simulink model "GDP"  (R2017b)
settings: Solver=FixedStepDiscrete  StartTime=0.0  StopTime=10.0  FixedStep=0.01  RelTol=1e-3  EnableMultiTasking=on
undefined symbols (not defined in the file): ASWTYPE_FALSE, ASWTYPE_TRUE, CcGDP_DCCANBusOffFltTi_ms, Enum_DCCDCConnSt, Enum_LDPCC2St, GDP_CONST1_NUMB, GDP_RUNTIME_MS
libraries: AIWAYS_Powertrain_BMS_lib x68
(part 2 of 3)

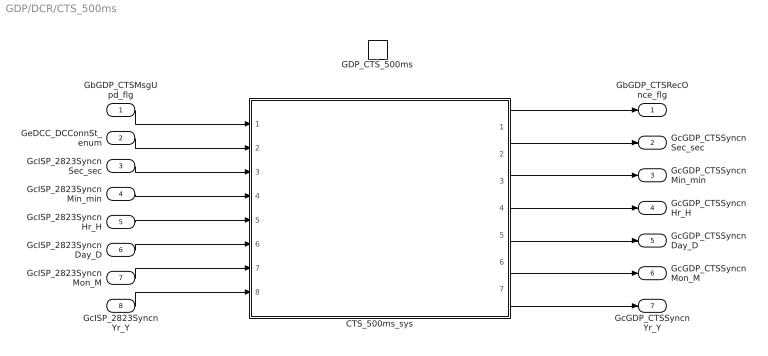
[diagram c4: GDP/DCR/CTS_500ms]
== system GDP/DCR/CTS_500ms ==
  GbGDP_CTSMsgUpd_flg : Inport
  GeDCC_DCConnSt_enum : Inport  Port=2
  GcISP_2823SyncnSec_sec : Inport  Port=3
  GcISP_2823SyncnMin_min : Inport  Port=4
  GcISP_2823SyncnHr_H : Inport  Port=5
  GcISP_2823SyncnDay_D : Inport  Port=6
  GcISP_2823SyncnMon_M : Inport  Port=7
  GcISP_2823SyncnYr_Y : Inport  Port=8
  GDP_CTS_500ms : TriggerPort  TriggerType=function-call  VariantControl=(inherit)
  CTS_500ms_sys : Subsystem
  GbGDP_CTSRecOnce_flg : Outport
  GcGDP_CTSSyncnSec_sec : Outport  Port=2
  GcGDP_CTSSyncnMin_min : Outport  Port=3
  GcGDP_CTSSyncnHr_H : Outport  Port=4
  GcGDP_CTSSyncnDay_D : Outport  Port=5
  GcGDP_CTSSyncnMon_M : Outport  Port=6
  GcGDP_CTSSyncnYr_Y : Outport  Port=7
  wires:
  GbGDP_CTSMsgUpd_flg/1 -> CTS_500ms_sys/1(GbGDP_CTSMsgUpd_flg)
  GeDCC_DCConnSt_enum/1 -> CTS_500ms_sys/2(GeDCC_DCConnSt_enum)
  GcISP_2823SyncnSec_sec/1 -> CTS_500ms_sys/3(GcISP_2823SyncnSec_sec)
  GcISP_2823SyncnMin_min/1 -> CTS_500ms_sys/4(GcISP_2823SyncnMin_min)
  GcISP_2823SyncnHr_H/1 -> CTS_500ms_sys/5(GcISP_2823SyncnHr_H)
  GcISP_2823SyncnDay_D/1 -> CTS_500ms_sys/6(GcISP_2823SyncnDay_D)
  GcISP_2823SyncnMon_M/1 -> CTS_500ms_sys/7(GcISP_2823SyncnMon_M)
  GcISP_2823SyncnYr_Y/1 -> CTS_500ms_sys/8(GcISP_2823SyncnYr_Y)
  CTS_500ms_sys/1(GbGDP_CTSRecOnce_flg) -> GbGDP_CTSRecOnce_flg/1
  CTS_500ms_sys/2(GcGDP_CTSSyncnSec_sec) -> GcGDP_CTSSyncnSec_sec/1
  CTS_500ms_sys/3(GcGDP_CTSSyncnMin_min) -> GcGDP_CTSSyncnMin_min/1
  CTS_500ms_sys/4(GcGDP_CTSSyncnHr_H) -> GcGDP_CTSSyncnHr_H/1
  CTS_500ms_sys/5(GcGDP_CTSSyncnDay_D) -> GcGDP_CTSSyncnDay_D/1
  CTS_500ms_sys/6(GcGDP_CTSSyncnMon_M) -> GcGDP_CTSSyncnMon_M/1
  CTS_500ms_sys/7(GcGDP_CTSSyncnYr_Y) -> GcGDP_CTSSyncnYr_Y/1

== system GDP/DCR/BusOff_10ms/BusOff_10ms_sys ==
  GbISP_DCCANBusOffFlt_flg : Inport
  GbISP_DCChrgCanNetStatus_flg : Inport  Port=2
  Constant : Constant  Value=GDP_RUNTIME_MS
  Constant1 : Constant  Value=CcGDP_DCCANBusOffFltTi_ms
  Delay : AIWAYS_Powertrain_BMS_lib/Debounce & Delay/BMSDelay
  GDP_GbISP_DCCANBusOffFlt_flg : AIWAYS_Powertrain_BMS_lib/Signals/OverWrite  OverWrite_Value=CbGDP_DCCANBusOffFltOvr_flg  OverWrite_flag=CbGDP_DCCANBusOffFltOvrSwt_flg
  Logical Operator : Logic  AllPortsSameDT=off  OutDataTypeStr=boolean
  GbGDP_DCCANBusOffFlt_flg : Outport
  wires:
  GDP_GbISP_DCCANBusOffFlt_flg/1 -> GbGDP_DCCANBusOffFlt_flg/1  "GbGDP_DCCANBusOffFlt_flg"
  Constant/1 -> Delay/2
  Constant1/1 -> Delay/3
  Delay/1 -> GDP_GbISP_DCCANBusOffFlt_flg/1
  GbISP_DCCANBusOffFlt_flg/1 -> Logical Operator/1  "GbISP_DCCANBusOffFlt_flg"
  GbISP_DCChrgCanNetStatus_flg/1 -> Logical Operator/2  "GbISP_DCChrgCanNetStatus_flg"
  Logical Operator/1 -> Delay/1

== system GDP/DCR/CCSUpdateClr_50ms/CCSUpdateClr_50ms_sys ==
  Constant : Constant  Value=ASWTYPE_FALSE
  GDP_GbGDP_CCSMsgUpd_flg : AIWAYS_Powertrain_BMS_lib/Signals/OverWrite  OverWrite_Value=CbGDP_CCSMsgUpdOvr_flg  OverWrite_flag=CbGDP_CCSMsgUpdOvrSwt_flg
  Signal Conversion1 : SignalConversion  OverrideOpt=off
  GbGDP_CCSMsgUpd_flg : Outport
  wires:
  Constant/1 -> Signal Conversion1/1
  GDP_GbGDP_CCSMsgUpd_flg/1 -> GbGDP_CCSMsgUpd_flg/1  "GbGDP_CCSMsgUpd_flg"
  Signal Conversion1/1 -> GDP_GbGDP_CCSMsgUpd_flg/1

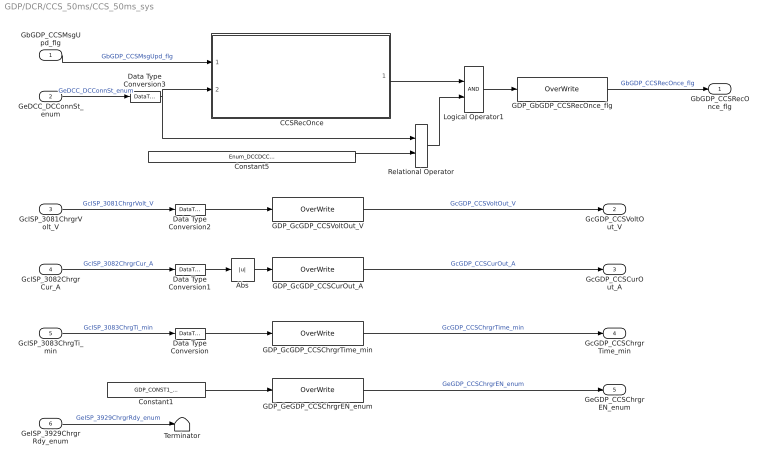
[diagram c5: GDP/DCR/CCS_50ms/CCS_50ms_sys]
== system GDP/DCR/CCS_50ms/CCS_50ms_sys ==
  GbGDP_CCSMsgUpd_flg : Inport
  GeDCC_DCConnSt_enum : Inport  Port=2
  GcISP_3081ChrgrVolt_V : Inport  Port=3
  GcISP_3082ChrgrCur_A : Inport  Port=4
  GcISP_3083ChrgTi_min : Inport  Port=5
  GeISP_3929ChrgrRdy_enum : Inport  Port=6
  " CCSRecOnce" : Subsystem
  Abs : Abs
  Constant1 : Constant  Value=GDP_CONST1_NUMB
  Constant5 : Constant  Value=Enum_DCCDCConnSt.Enum_DCCDCConnSt_Chrging
  Data Type Conversion{,1..3} (4 alike) : DataTypeConversion
  GDP_GbGDP_CCSRecOnce_flg : AIWAYS_Powertrain_BMS_lib/Signals/OverWrite  OverWrite_Value=CbGDP_CCSRecOnceOvr_flg  OverWrite_flag=CbGDP_CCSRecOnceOvrSwt_flg
  GDP_GcGDP_CCSChrgrTime_min : AIWAYS_Powertrain_BMS_lib/Signals/OverWrite  OverWrite_Value=CcGDP_CCSChrgrTimeOvr_min  OverWrite_flag=CbGDP_CCSChrgrTimeOvrSwt_flg
  GDP_GcGDP_CCSCurOut_A : AIWAYS_Powertrain_BMS_lib/Signals/OverWrite  OverWrite_Value=CcGDP_CCSCurOutOvr_A  OverWrite_flag=CbGDP_CCSCurOutOvrSwt_flg
  GDP_GcGDP_CCSVoltOut_V : AIWAYS_Powertrain_BMS_lib/Signals/OverWrite  OverWrite_Value=CcGDP_CCSVoltOutOvr_V  OverWrite_flag=CbGDP_CCSVoltOutOvrSwt_flg
  GDP_GeGDP_CCSChrgrEN_enum : AIWAYS_Powertrain_BMS_lib/Signals/OverWrite  OverWrite_Value=CeGDP_CCSChrgrENOvr_enum  OverWrite_flag=CbGDP_CCSChrgrENOvrSwt_flg
  Logical Operator1 : Logic  AllPortsSameDT=off  OutDataTypeStr=boolean
  Relational Operator : RelationalOperator  Operator===  OutDataTypeStr=boolean
  Terminator : Terminator
  GbGDP_CCSRecOnce_flg : Outport
  GcGDP_CCSVoltOut_V : Outport  Port=2
  GcGDP_CCSCurOut_A : Outport  Port=3
  GcGDP_CCSChrgrTime_min : Outport  Port=4
  GeGDP_CCSChrgrEN_enum : Outport  Port=5
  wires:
  GbGDP_CCSMsgUpd_flg/1 -> " CCSRecOnce"/1(GbGDP_CCSMsgUpd_flg)  "GbGDP_CCSMsgUpd_flg"
  Relational Operator/1 -> Logical Operator1/2
  Constant5/1 -> Relational Operator/2
  " CCSRecOnce"/1(LbGDP_CCSRecOnce_flg) -> Logical Operator1/1
  Logical Operator1/1 -> GDP_GbGDP_CCSRecOnce_flg/1
  GeDCC_DCConnSt_enum/1 -> Data Type Conversion3/1  "GeDCC_DCConnSt_enum"
  GcISP_3081ChrgrVolt_V/1 -> Data Type Conversion2/1  "GcISP_3081ChrgrVolt_V"
  GcISP_3082ChrgrCur_A/1 -> Data Type Conversion1/1  "GcISP_3082ChrgrCur_A"
  GcISP_3083ChrgTi_min/1 -> Data Type Conversion/1  "GcISP_3083ChrgTi_min"
  GDP_GbGDP_CCSRecOnce_flg/1 -> GbGDP_CCSRecOnce_flg/1  "GbGDP_CCSRecOnce_flg"
  GDP_GcGDP_CCSVoltOut_V/1 -> GcGDP_CCSVoltOut_V/1  "GcGDP_CCSVoltOut_V"
  GDP_GcGDP_CCSCurOut_A/1 -> GcGDP_CCSCurOut_A/1  "GcGDP_CCSCurOut_A"
  GDP_GcGDP_CCSChrgrTime_min/1 -> GcGDP_CCSChrgrTime_min/1  "GcGDP_CCSChrgrTime_min"
  GDP_GeGDP_CCSChrgrEN_enum/1 -> GeGDP_CCSChrgrEN_enum/1  "GeGDP_CCSChrgrEN_enum"
  Data Type Conversion/1 -> GDP_GcGDP_CCSChrgrTime_min/1
  Data Type Conversion1/1 -> Abs/1
  Data Type Conversion2/1 -> GDP_GcGDP_CCSVoltOut_V/1
  Abs/1 -> GDP_GcGDP_CCSCurOut_A/1
  GeISP_3929ChrgrRdy_enum/1 -> Terminator/1  "GeISP_3929ChrgrRdy_enum"
  Constant1/1 -> GDP_GeGDP_CCSChrgrEN_enum/1
  Data Type Conversion3/1 -> " CCSRecOnce"/2(GeDCC_DCConnSt_enum), Relational Operator/1

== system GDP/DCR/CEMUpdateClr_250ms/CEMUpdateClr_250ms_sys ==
  Constant : Constant  Value=ASWTYPE_FALSE
  GDP_GbGDP_CEMMsgUpd_flg : AIWAYS_Powertrain_BMS_lib/Signals/OverWrite  OverWrite_Value=CbGDP_CEMMsgUpdOvr_flg  OverWrite_flag=CbGDP_CEMMsgUpdOvrSwt_flg
  Signal Conversion1 : SignalConversion  OverrideOpt=off
  GbGDP_CEMMsgUpd_flg : Outport
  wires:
  Constant/1 -> Signal Conversion1/1
  Signal Conversion1/1 -> GDP_GbGDP_CEMMsgUpd_flg/1
  GDP_GbGDP_CEMMsgUpd_flg/1 -> GbGDP_CEMMsgUpd_flg/1  "GbGDP_CEMMsgUpd_flg"

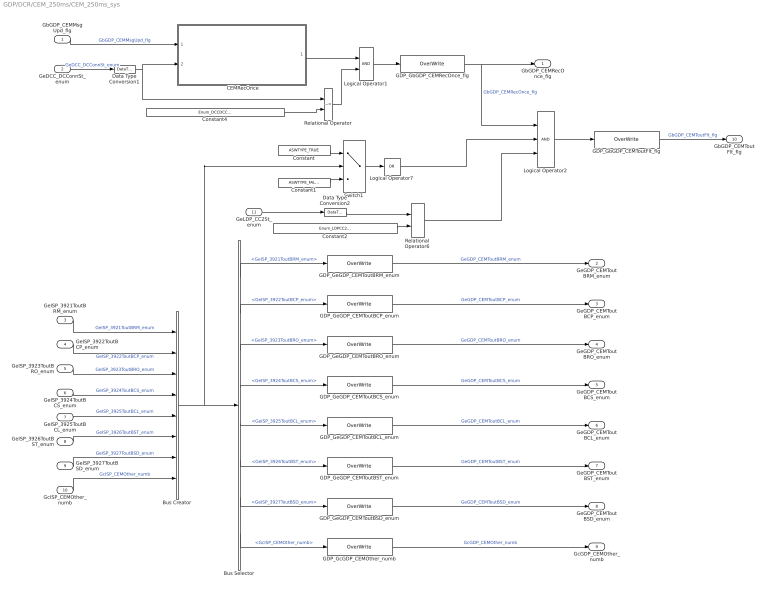
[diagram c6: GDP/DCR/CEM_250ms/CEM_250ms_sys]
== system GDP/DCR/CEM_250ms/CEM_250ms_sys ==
  GbGDP_CEMMsgUpd_flg : Inport
  GeDCC_DCConnSt_enum : Inport  Port=2
  GeISP_3921ToutBRM_enum : Inport  Port=3
  GeISP_3922ToutBCP_enum : Inport  Port=4
  GeISP_3923ToutBRO_enum : Inport  Port=5
  GeISP_3924ToutBCS_enum : Inport  Port=6
  GeISP_3925ToutBCL_enum : Inport  Port=7
  GeISP_3926ToutBST_enum : Inport  Port=8
  GeISP_3927ToutBSD_enum : Inport  Port=9
  GcISP_CEMOther_numb : Inport  Port=10
  GeLDP_CC2St_enum : Inport  Port=11
  " CEMRecOnce" : Subsystem
  Bus Creator : BusCreator  Inputs=8
  Bus Selector : BusSelector  OutputSignals=GeISP_3921ToutBRM_enum,GeISP_3922ToutBCP_enum,GeISP_3923ToutBRO_enum,GeISP_3924ToutBCS_enum,GeISP_3925ToutBCL_enum,GeISP_3926ToutBST_enum,GeISP_3927ToutBSD_enum,GcISP_CEMOther_numb
  Constant : Constant  Value=ASWTYPE_TRUE
  Constant1 : Constant  Value=ASWTYPE_FALSE
  Constant2 : Constant  Value=Enum_LDPCC2St.Enum_LDPCC2St_Connect
  Constant4 : Constant  Value=Enum_DCCDCConnSt.Enum_DCCDCConnSt_Default
  Data Type Conversion1 : DataTypeConversion
  Data Type Conversion2 : DataTypeConversion
  GDP_GbGDP_CEMRecOnce_flg : AIWAYS_Powertrain_BMS_lib/Signals/OverWrite  OverWrite_Value=CbGDP_CEMRecOnceOvr_flg  OverWrite_flag=CbGDP_CEMRecOnceOvrSwt_flg
  GDP_GbGDP_CEMToutFlt_flg : AIWAYS_Powertrain_BMS_lib/Signals/OverWrite  OverWrite_Value=CbGDP_CEMToutFltOvr_flg  OverWrite_flag=CbGDP_CEMToutFltOvrSwt_flg
  GDP_GcGDP_CEMOther_numb : AIWAYS_Powertrain_BMS_lib/Signals/OverWrite  OverWrite_Value=CcGDP_CEMOtherOvr_numb  OverWrite_flag=CbGDP_CEMOtherOvrSwt_flg
  GDP_GeGDP_CEMToutBCL_enum : AIWAYS_Powertrain_BMS_lib/Signals/OverWrite  OverWrite_Value=CeGDP_CEMToutBCLOvr_enum  OverWrite_flag=CbGDP_CEMToutBCLOvrSwt_flg
  GDP_GeGDP_CEMToutBCP_enum : AIWAYS_Powertrain_BMS_lib/Signals/OverWrite  OverWrite_Value=CeGDP_CEMToutBCPOvr_enum  OverWrite_flag=CbGDP_CEMToutBCPOvrSwt_flg
  GDP_GeGDP_CEMToutBCS_enum : AIWAYS_Powertrain_BMS_lib/Signals/OverWrite  OverWrite_Value=CeGDP_CEMToutBCSOvr_enum  OverWrite_flag=CbGDP_CEMToutBCSOvrSwt_flg
  GDP_GeGDP_CEMToutBRM_enum : AIWAYS_Powertrain_BMS_lib/Signals/OverWrite  OverWrite_Value=CeGDP_CEMToutBRMOvr_enum  OverWrite_flag=CbGDP_CEMToutBRMOvrSwt_flg
  GDP_GeGDP_CEMToutBRO_enum : AIWAYS_Powertrain_BMS_lib/Signals/OverWrite  OverWrite_Value=CeGDP_CEMToutBROOvr_enum  OverWrite_flag=CbGDP_CEMToutBROOvrSwt_flg
  GDP_GeGDP_CEMToutBSD_enum : AIWAYS_Powertrain_BMS_lib/Signals/OverWrite  OverWrite_Value=CeGDP_CEMToutBSDOvr_enum  OverWrite_flag=CbGDP_CEMToutBSDOvrSwt_flg
  GDP_GeGDP_CEMToutBST_enum : AIWAYS_Powertrain_BMS_lib/Signals/OverWrite  OverWrite_Value=CeGDP_CEMToutBSTOvr_enum  OverWrite_flag=CbGDP_CEMToutBSTOvrSwt_flg
  Logical Operator1 : Logic  AllPortsSameDT=off  OutDataTypeStr=boolean
  Logical Operator2 : Logic  Inputs=3  AllPortsSameDT=off  OutDataTypeStr=boolean
  Logical Operator7 : Logic  Operator=OR  Inputs=1  AllPortsSameDT=off  OutDataTypeStr=boolean
  Relational Operator : RelationalOperator  Operator=~=  OutDataTypeStr=boolean
  Relational Operator6 : RelationalOperator  Operator===  OutDataTypeStr=boolean
  Switch1 : Switch  Criteria=u2 ~= 0
  GbGDP_CEMRecOnce_flg : Outport
  GeGDP_CEMToutBRM_enum : Outport  Port=2
  GeGDP_CEMToutBCP_enum : Outport  Port=3
  GeGDP_CEMToutBRO_enum : Outport  Port=4
  GeGDP_CEMToutBCS_enum : Outport  Port=5
  GeGDP_CEMToutBCL_enum : Outport  Port=6
  GeGDP_CEMToutBST_enum : Outport  Port=7
  GeGDP_CEMToutBSD_enum : Outport  Port=8
  GcGDP_CEMOther_numb : Outport  Port=9
  GbGDP_CEMToutFlt_flg : Outport  Port=10
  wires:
  GbGDP_CEMMsgUpd_flg/1 -> " CEMRecOnce"/1(GbGDP_CEMMsgUpd_flg)  "GbGDP_CEMMsgUpd_flg"
  Relational Operator/1 -> Logical Operator1/2
  Constant4/1 -> Relational Operator/2
  " CEMRecOnce"/1(LbGDP_CEMRecOnce_flg) -> Logical Operator1/1
  Logical Operator1/1 -> GDP_GbGDP_CEMRecOnce_flg/1
  GeDCC_DCConnSt_enum/1 -> Data Type Conversion1/1  "GeDCC_DCConnSt_enum"
  GDP_GbGDP_CEMRecOnce_flg/1 -> Logical Operator2/1, GbGDP_CEMRecOnce_flg/1  "GbGDP_CEMRecOnce_flg"
  GDP_GeGDP_CEMToutBRM_enum/1 -> GeGDP_CEMToutBRM_enum/1  "GeGDP_CEMToutBRM_enum"
  GDP_GeGDP_CEMToutBCP_enum/1 -> GeGDP_CEMToutBCP_enum/1  "GeGDP_CEMToutBCP_enum"
  GDP_GeGDP_CEMToutBRO_enum/1 -> GeGDP_CEMToutBRO_enum/1  "GeGDP_CEMToutBRO_enum"
  GDP_GeGDP_CEMToutBCS_enum/1 -> GeGDP_CEMToutBCS_enum/1  "GeGDP_CEMToutBCS_enum"
  GDP_GeGDP_CEMToutBCL_enum/1 -> GeGDP_CEMToutBCL_enum/1  "GeGDP_CEMToutBCL_enum"
  GDP_GeGDP_CEMToutBST_enum/1 -> GeGDP_CEMToutBST_enum/1  "GeGDP_CEMToutBST_enum"
  GDP_GeGDP_CEMToutBSD_enum/1 -> GeGDP_CEMToutBSD_enum/1  "GeGDP_CEMToutBSD_enum"
  GDP_GcGDP_CEMOther_numb/1 -> GcGDP_CEMOther_numb/1  "GcGDP_CEMOther_numb"
  GeISP_3921ToutBRM_enum/1 -> Bus Creator/1  "GeISP_3921ToutBRM_enum"
  GeISP_3922ToutBCP_enum/1 -> Bus Creator/2  "GeISP_3922ToutBCP_enum"
  GeISP_3923ToutBRO_enum/1 -> Bus Creator/3  "GeISP_3923ToutBRO_enum"
  GeISP_3924ToutBCS_enum/1 -> Bus Creator/4  "GeISP_3924ToutBCS_enum"
  GeISP_3925ToutBCL_enum/1 -> Bus Creator/5  "GeISP_3925ToutBCL_enum"
  GeISP_3926ToutBST_enum/1 -> Bus Creator/6  "GeISP_3926ToutBST_enum"
  GeISP_3927ToutBSD_enum/1 -> Bus Creator/7  "GeISP_3927ToutBSD_enum"
  GcISP_CEMOther_numb/1 -> Bus Creator/8  "GcISP_CEMOther_numb"
  Bus Selector/1 -> GDP_GeGDP_CEMToutBRM_enum/1  "<GeISP_3921ToutBRM_enum>"
  Bus Selector/2 -> GDP_GeGDP_CEMToutBCP_enum/1  "<GeISP_3922ToutBCP_enum>"
  Bus Selector/3 -> GDP_GeGDP_CEMToutBRO_enum/1  "<GeISP_3923ToutBRO_enum>"
  Bus Selector/4 -> GDP_GeGDP_CEMToutBCS_enum/1  "<GeISP_3924ToutBCS_enum>"
  Bus Selector/5 -> GDP_GeGDP_CEMToutBCL_enum/1  "<GeISP_3925ToutBCL_enum>"
  Bus Selector/6 -> GDP_GeGDP_CEMToutBST_enum/1  "<GeISP_3926ToutBST_enum>"
  Bus Selector/7 -> GDP_GeGDP_CEMToutBSD_enum/1  "<GeISP_3927ToutBSD_enum>"
  Bus Selector/8 -> GDP_GcGDP_CEMOther_numb/1  "<GcISP_CEMOther_numb>"
  Constant1/1 -> Switch1/3
  Bus Creator/1 -> Bus Selector/1, Switch1/2
  Constant/1 -> Switch1/1
  Switch1/1 -> Logical Operator7/1
  GDP_GbGDP_CEMToutFlt_flg/1 -> GbGDP_CEMToutFlt_flg/1  "GbGDP_CEMToutFlt_flg"
  Data Type Conversion1/1 -> " CEMRecOnce"/2(GeDCC_DCConnSt_enum), Relational Operator/1
  GeLDP_CC2St_enum/1 -> Data Type Conversion2/1
  Constant2/1 -> Relational Operator6/2
  Data Type Conversion2/1 -> Relational Operator6/1
  Logical Operator2/1 -> GDP_GbGDP_CEMToutFlt_flg/1
  Logical Operator7/1 -> Logical Operator2/2
  Relational Operator6/1 -> Logical Operator2/3

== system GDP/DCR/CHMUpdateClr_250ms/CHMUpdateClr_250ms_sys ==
  Constant : Constant  Value=ASWTYPE_FALSE
  GDP_GbGDP_CHMMsgUpd_flg : AIWAYS_Powertrain_BMS_lib/Signals/OverWrite  OverWrite_Value=CbGDP_CHMMsgUpdOvr_flg  OverWrite_flag=CbGDP_CHMMsgUpdOvrSwt_flg
  Signal Conversion1 : SignalConversion  OverrideOpt=off
  GbGDP_CHMMsgUpd_flg : Outport
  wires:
  GDP_GbGDP_CHMMsgUpd_flg/1 -> GbGDP_CHMMsgUpd_flg/1  "GbGDP_CHMMsgUpd_flg"
  Signal Conversion1/1 -> GDP_GbGDP_CHMMsgUpd_flg/1
  Constant/1 -> Signal Conversion1/1

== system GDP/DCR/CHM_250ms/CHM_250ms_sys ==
  GbGDP_CHMMsgUpd_flg : Inport
  GeDCC_DCConnSt_enum : Inport  Port=2
  GcISP_2600ChrgrVer_numb : Inport  Port=3
  GbLDP_DC12VSply_flg : Inport  Port=4
  " CHMRecOnce" : Subsystem
  Constant1 : Constant  Value=Enum_DCCDCConnSt.Enum_DCCDCConnSt_HandShake
  Constant4 : Constant  Value=Enum_DCCDCConnSt.Enum_DCCDCConnSt_Default
  Data Type Conversion2 : DataTypeConversion
  GDP_GbGDP_CHMRecOnce_flg : AIWAYS_Powertrain_BMS_lib/Signals/OverWrite  OverWrite_Value=CbGDP_CHMRecOnceOvr_flg  OverWrite_flag=CbGDP_CHMRecOnceOvrSwt_flg
  GDP_GcGDP_CHM2600ChrgrVer_numb : AIWAYS_Powertrain_BMS_lib/Signals/OverWrite  OverWrite_Value=CcGDP_CHM2600ChrgrVerOvr_numb  OverWrite_flag=CbGDP_CHM2600ChrgrVerOvrSwt_flg
  Logical Operator : Logic  Operator=OR  AllPortsSameDT=off  OutDataTypeStr=boolean
  Logical Operator1 : Logic  AllPortsSameDT=off  OutDataTypeStr=boolean
  Logical Operator2 : Logic  AllPortsSameDT=off  OutDataTypeStr=boolean
  Relational Operator : RelationalOperator  Operator===  OutDataTypeStr=boolean
  Relational Operator1 : RelationalOperator  Operator===  OutDataTypeStr=boolean
  GbGDP_CHMRecOnce_flg : Outport
  GcGDP_CHM2600ChrgrVer_numb : Outport  Port=2
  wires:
  GbGDP_CHMMsgUpd_flg/1 -> " CHMRecOnce"/1(GbGDP_CHMMsgUpd_flg)  "GbGDP_CHMMsgUpd_flg"
  GeDCC_DCConnSt_enum/1 -> Data Type Conversion2/1  "GeDCC_DCConnSt_enum"
  Constant1/1 -> Relational Operator1/2
  Constant4/1 -> Relational Operator/2
  Relational Operator/1 -> Logical Operator/1
  Relational Operator1/1 -> Logical Operator/2
  " CHMRecOnce"/1(LbGDP_CHMRecOnce_flg) -> Logical Operator1/1
  Logical Operator1/1 -> GDP_GbGDP_CHMRecOnce_flg/1
  GcISP_2600ChrgrVer_numb/1 -> GDP_GcGDP_CHM2600ChrgrVer_numb/1  "GcISP_2600ChrgrVer_numb"
  GDP_GcGDP_CHM2600ChrgrVer_numb/1 -> GcGDP_CHM2600ChrgrVer_numb/1  "GcGDP_CHM2600ChrgrVer_numb"
  GDP_GbGDP_CHMRecOnce_flg/1 -> GbGDP_CHMRecOnce_flg/1  "GbGDP_CHMRecOnce_flg"
  Data Type Conversion2/1 -> " CHMRecOnce"/3(GeDCC_DCConnSt_enum), Relational Operator/1, Relational Operator1/1
  GbLDP_DC12VSply_flg/1 -> Logical Operator2/2, " CHMRecOnce"/2(GbLDP_DC12VSply_flg)  "GbLDP_DC12VSply_flg"
  Logical Operator/1 -> Logical Operator2/1
  Logical Operator2/1 -> Logical Operator1/2

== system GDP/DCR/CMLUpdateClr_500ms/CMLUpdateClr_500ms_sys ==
  Constant : Constant  Value=ASWTYPE_FALSE
  GDP_GbGDP_CMLMsgUpd_flg : AIWAYS_Powertrain_BMS_lib/Signals/OverWrite  OverWrite_Value=CbGDP_CMLMsgUpdOvr_flg  OverWrite_flag=CbGDP_CMLMsgUpdOvrSwt_flg
  Signal Conversion1 : SignalConversion  OverrideOpt=off
  GbGDP_CMLMsgUpd_flg : Outport
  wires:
  GDP_GbGDP_CMLMsgUpd_flg/1 -> GbGDP_CMLMsgUpd_flg/1  "GbGDP_CMLMsgUpd_flg"
  Signal Conversion1/1 -> GDP_GbGDP_CMLMsgUpd_flg/1
  Constant/1 -> Signal Conversion1/1

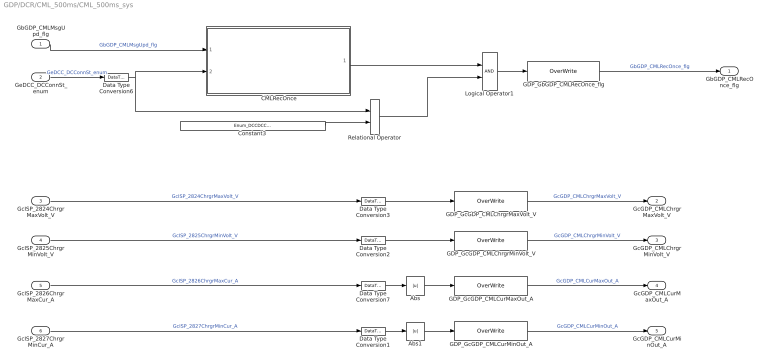
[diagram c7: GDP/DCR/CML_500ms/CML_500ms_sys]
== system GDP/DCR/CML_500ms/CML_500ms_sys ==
  GbGDP_CMLMsgUpd_flg : Inport
  GeDCC_DCConnSt_enum : Inport  Port=2
  GcISP_2824ChrgrMaxVolt_V : Inport  Port=3
  GcISP_2825ChrgrMinVolt_V : Inport  Port=4
  GcISP_2826ChrgrMaxCur_A : Inport  Port=5
  GcISP_2827ChrgrMinCur_A : Inport  Port=6
  " CMLRecOnce" : Subsystem
  Abs : Abs
  Abs1 : Abs
  Constant3 : Constant  Value=Enum_DCCDCConnSt.Enum_DCCDCConnSt_CFG
  Data Type Conversion{1..3,6..7} (5 alike) : DataTypeConversion
  GDP_GbGDP_CMLRecOnce_flg : AIWAYS_Powertrain_BMS_lib/Signals/OverWrite  OverWrite_Value=CbGDP_CMLRecOnceOvr_flg  OverWrite_flag=CbGDP_CMLRecOnceOvrSwt_flg
  GDP_GcGDP_CMLChrgrMaxVolt_V : AIWAYS_Powertrain_BMS_lib/Signals/OverWrite  OverWrite_Value=CcGDP_CMLChrgrMaxVoltOvr_V  OverWrite_flag=CbGDP_CMLChrgrMaxVoltOvrSwt_flg
  GDP_GcGDP_CMLChrgrMinVolt_V : AIWAYS_Powertrain_BMS_lib/Signals/OverWrite  OverWrite_Value=CcGDP_CMLChrgrMinVoltOvr_V  OverWrite_flag=CbGDP_CMLChrgrMinVoltOvrSwt_flg
  GDP_GcGDP_CMLCurMaxOut_A : AIWAYS_Powertrain_BMS_lib/Signals/OverWrite  OverWrite_Value=CcGDP_CMLCurMaxOutOvr_A  OverWrite_flag=CbGDP_CMLCurMaxOutOvrSwt_flg
  GDP_GcGDP_CMLCurMinOut_A : AIWAYS_Powertrain_BMS_lib/Signals/OverWrite  OverWrite_Value=CcGDP_CMLCurMinOutOvr_A  OverWrite_flag=CbGDP_CMLCurMinOutOvrSwt_flg
  Logical Operator1 : Logic  AllPortsSameDT=off  OutDataTypeStr=boolean
  Relational Operator : RelationalOperator  Operator===  OutDataTypeStr=boolean
  GbGDP_CMLRecOnce_flg : Outport
  GcGDP_CMLChrgrMaxVolt_V : Outport  Port=2
  GcGDP_CMLChrgrMinVolt_V : Outport  Port=3
  GcGDP_CMLCurMaxOut_A : Outport  Port=4
  GcGDP_CMLCurMinOut_A : Outport  Port=5
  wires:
  GbGDP_CMLMsgUpd_flg/1 -> " CMLRecOnce"/1(GbGDP_CMLMsgUpd_flg)  "GbGDP_CMLMsgUpd_flg"
  Constant3/1 -> Relational Operator/2
  " CMLRecOnce"/1(LbGDP_CMLRecOnce_flg) -> Logical Operator1/1
  Logical Operator1/1 -> GDP_GbGDP_CMLRecOnce_flg/1
  GeDCC_DCConnSt_enum/1 -> Data Type Conversion6/1  "GeDCC_DCConnSt_enum"
  GcISP_2824ChrgrMaxVolt_V/1 -> Data Type Conversion3/1  "GcISP_2824ChrgrMaxVolt_V"
  GcISP_2825ChrgrMinVolt_V/1 -> Data Type Conversion2/1  "GcISP_2825ChrgrMinVolt_V"
  GcISP_2826ChrgrMaxCur_A/1 -> Data Type Conversion7/1  "GcISP_2826ChrgrMaxCur_A"
  GcISP_2827ChrgrMinCur_A/1 -> Data Type Conversion1/1  "GcISP_2827ChrgrMinCur_A"
  GDP_GcGDP_CMLChrgrMaxVolt_V/1 -> GcGDP_CMLChrgrMaxVolt_V/1  "GcGDP_CMLChrgrMaxVolt_V"
  GDP_GcGDP_CMLChrgrMinVolt_V/1 -> GcGDP_CMLChrgrMinVolt_V/1  "GcGDP_CMLChrgrMinVolt_V"
  GDP_GcGDP_CMLCurMaxOut_A/1 -> GcGDP_CMLCurMaxOut_A/1  "GcGDP_CMLCurMaxOut_A"
  GDP_GcGDP_CMLCurMinOut_A/1 -> GcGDP_CMLCurMinOut_A/1  "GcGDP_CMLCurMinOut_A"
  GDP_GbGDP_CMLRecOnce_flg/1 -> GbGDP_CMLRecOnce_flg/1  "GbGDP_CMLRecOnce_flg"
  Data Type Conversion1/1 -> Abs1/1
  Data Type Conversion7/1 -> Abs/1
  Data Type Conversion2/1 -> GDP_GcGDP_CMLChrgrMinVolt_V/1
  Data Type Conversion3/1 -> GDP_GcGDP_CMLChrgrMaxVolt_V/1
  Abs/1 -> GDP_GcGDP_CMLCurMaxOut_A/1
  Abs1/1 -> GDP_GcGDP_CMLCurMinOut_A/1
  Relational Operator/1 -> Logical Operator1/2
  Data Type Conversion6/1 -> " CMLRecOnce"/2(GeDCC_DCConnSt_enum), Relational Operator/1

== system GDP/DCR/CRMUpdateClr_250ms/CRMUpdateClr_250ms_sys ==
  Constant : Constant  Value=ASWTYPE_FALSE
  GDP_GbGDP_CRMMsgUpd_flg : AIWAYS_Powertrain_BMS_lib/Signals/OverWrite  OverWrite_Value=CbGDP_CRMMsgUpdOvr_flg  OverWrite_flag=CbGDP_CRMMsgUpdOvrSwt_flg
  Signal Conversion1 : SignalConversion  OverrideOpt=off
  GbGDP_CRMMsgUpd_flg : Outport
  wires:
  GDP_GbGDP_CRMMsgUpd_flg/1 -> GbGDP_CRMMsgUpd_flg/1  "GbGDP_CRMMsgUpd_flg"
  Signal Conversion1/1 -> GDP_GbGDP_CRMMsgUpd_flg/1
  Constant/1 -> Signal Conversion1/1

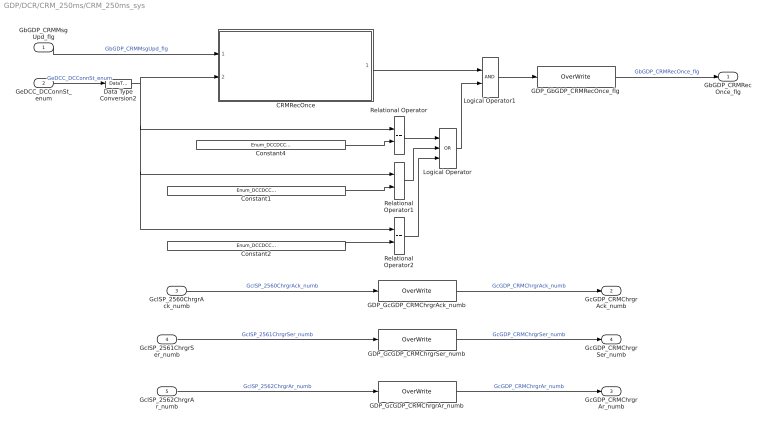
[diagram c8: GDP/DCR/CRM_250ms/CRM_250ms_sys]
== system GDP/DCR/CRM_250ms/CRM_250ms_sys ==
  GbGDP_CRMMsgUpd_flg : Inport
  GeDCC_DCConnSt_enum : Inport  Port=2
  GcISP_2560ChrgrAck_numb : Inport  Port=3
  GcISP_2561ChrgrSer_numb : Inport  Port=4
  GcISP_2562ChrgrAr_numb : Inport  Port=5
  " CRMRecOnce" : Subsystem
  Constant1 : Constant  Value=Enum_DCCDCConnSt.Enum_DCCDCConnSt_HandShake
  Constant2 : Constant  Value=Enum_DCCDCConnSt.Enum_DCCDCConnSt_CommTout
  Constant4 : Constant  Value=Enum_DCCDCConnSt.Enum_DCCDCConnSt_ID
  Data Type Conversion2 : DataTypeConversion
  GDP_GbGDP_CRMRecOnce_flg : AIWAYS_Powertrain_BMS_lib/Signals/OverWrite  OverWrite_Value=CbGDP_CRMRecOnceOvr_flg  OverWrite_flag=CbGDP_CRMRecOnceOvrSwt_flg
  GDP_GcGDP_CRMChrgrAck_numb : AIWAYS_Powertrain_BMS_lib/Signals/OverWrite  OverWrite_Value=CcGDP_CRMChrgrAckOvr_numb  OverWrite_flag=CbGDP_CRMChrgrAckOvrSwt_flg
  GDP_GcGDP_CRMChrgrAr_numb : AIWAYS_Powertrain_BMS_lib/Signals/OverWrite  OverWrite_Value=CcGDP_CRMChrgrArOvr_numb  OverWrite_flag=CbGDP_CRMChrgrArOvrSwt_flg
  GDP_GcGDP_CRMChrgrSer_numb : AIWAYS_Powertrain_BMS_lib/Signals/OverWrite  OverWrite_Value=CcGDP_CRMChrgrSerOvr_numb  OverWrite_flag=CbGDP_CRMChrgrSerOvrSwt_flg
  Logical Operator : Logic  Operator=OR  Inputs=3  AllPortsSameDT=off  OutDataTypeStr=boolean
  Logical Operator1 : Logic  AllPortsSameDT=off  OutDataTypeStr=boolean
  Relational Operator : RelationalOperator  Operator===  OutDataTypeStr=boolean
  Relational Operator1 : RelationalOperator  Operator===  OutDataTypeStr=boolean
  Relational Operator2 : RelationalOperator  Operator===  OutDataTypeStr=boolean
  GbGDP_CRMRecOnce_flg : Outport
  GcGDP_CRMChrgrAck_numb : Outport  Port=2
  GcGDP_CRMChrgrAr_numb : Outport  Port=3
  GcGDP_CRMChrgrSer_numb : Outport  Port=4
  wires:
  GbGDP_CRMMsgUpd_flg/1 -> " CRMRecOnce"/1(GbGDP_CRMMsgUpd_flg)  "GbGDP_CRMMsgUpd_flg"
  Logical Operator/1 -> Logical Operator1/2
  Constant1/1 -> Relational Operator1/2
  Constant4/1 -> Relational Operator/2
  Relational Operator/1 -> Logical Operator/1
  Relational Operator1/1 -> Logical Operator/2
  " CRMRecOnce"/1(LbGDP_CRMRecOnce_flg) -> Logical Operator1/1
  Logical Operator1/1 -> GDP_GbGDP_CRMRecOnce_flg/1
  GeDCC_DCConnSt_enum/1 -> Data Type Conversion2/1  "GeDCC_DCConnSt_enum"
  GDP_GbGDP_CRMRecOnce_flg/1 -> GbGDP_CRMRecOnce_flg/1  "GbGDP_CRMRecOnce_flg"
  GDP_GcGDP_CRMChrgrAck_numb/1 -> GcGDP_CRMChrgrAck_numb/1  "GcGDP_CRMChrgrAck_numb"
  GDP_GcGDP_CRMChrgrAr_numb/1 -> GcGDP_CRMChrgrAr_numb/1  "GcGDP_CRMChrgrAr_numb"
  GDP_GcGDP_CRMChrgrSer_numb/1 -> GcGDP_CRMChrgrSer_numb/1  "GcGDP_CRMChrgrSer_numb"
  Data Type Conversion2/1 -> " CRMRecOnce"/2(GeDCC_DCConnSt_enum), Relational Operator/1, Relational Operator2/1, Relational Operator1/1
  GcISP_2560ChrgrAck_numb/1 -> GDP_GcGDP_CRMChrgrAck_numb/1  "GcISP_2560ChrgrAck_numb"
  GcISP_2561ChrgrSer_numb/1 -> GDP_GcGDP_CRMChrgrSer_numb/1  "GcISP_2561ChrgrSer_numb"
  GcISP_2562ChrgrAr_numb/1 -> GDP_GcGDP_CRMChrgrAr_numb/1  "GcISP_2562ChrgrAr_numb"
  Constant2/1 -> Relational Operator2/2
  Relational Operator2/1 -> Logical Operator/3

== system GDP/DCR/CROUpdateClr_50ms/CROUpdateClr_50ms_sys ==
  Constant : Constant  Value=ASWTYPE_FALSE
  GDP_GbGDP_CROMsgUpd_flg : AIWAYS_Powertrain_BMS_lib/Signals/OverWrite  OverWrite_Value=CbGDP_CROMsgUpdOvr_flg  OverWrite_flag=CbGDP_CROMsgUpdOvrSwt_flg
  Signal Conversion1 : SignalConversion  OverrideOpt=off
  GbGDP_CROMsgUpd_flg : Outport
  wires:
  Signal Conversion1/1 -> GDP_GbGDP_CROMsgUpd_flg/1
  Constant/1 -> Signal Conversion1/1
  GDP_GbGDP_CROMsgUpd_flg/1 -> GbGDP_CROMsgUpd_flg/1  "GbGDP_CROMsgUpd_flg"

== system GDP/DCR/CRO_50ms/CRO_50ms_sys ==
  GbGDP_CROMsgUpd_flg : Inport
  GeDCC_DCConnSt_enum : Inport  Port=2
  GcISP_2830ChrgrRdy_numb : Inport  Port=3
  " CRORecOnce" : Subsystem
  Constant1 : Constant  Value=Enum_DCCDCConnSt.Enum_DCCDCConnSt_CFG
  Data Type Conversion1 : DataTypeConversion
  GDP_GbGDP_CRORecOnce_flg : AIWAYS_Powertrain_BMS_lib/Signals/OverWrite  OverWrite_Value=CbGDP_CRORecOnceOvr_flg  OverWrite_flag=CbGDP_CRORecOnceOvrSwt_flg
  GDP_GcGDP_CROChrgrRdy_numb : AIWAYS_Powertrain_BMS_lib/Signals/OverWrite  OverWrite_Value=CcGDP_CROChrgrRdyOvr_numb  OverWrite_flag=CbGDP_CROChrgrRdyOvrSwt_flg
  Logical Operator1 : Logic  AllPortsSameDT=off  OutDataTypeStr=boolean
  Relational Operator : RelationalOperator  Operator===  OutDataTypeStr=boolean
  GbGDP_CRORecOnce_flg : Outport
  GcGDP_CROChrgrRdy_numb : Outport  Port=2
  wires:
  GbGDP_CROMsgUpd_flg/1 -> " CRORecOnce"/1(GbGDP_CROMsgUpd_flg)  "GbGDP_CROMsgUpd_flg"
  Relational Operator/1 -> Logical Operator1/2
  Constant1/1 -> Relational Operator/2
  " CRORecOnce"/1(LbGDP_CRORecOnce_flg) -> Logical Operator1/1
  Logical Operator1/1 -> GDP_GbGDP_CRORecOnce_flg/1
  GeDCC_DCConnSt_enum/1 -> Data Type Conversion1/1  "GeDCC_DCConnSt_enum"
  GDP_GbGDP_CRORecOnce_flg/1 -> GbGDP_CRORecOnce_flg/1  "GbGDP_CRORecOnce_flg"
  GDP_GcGDP_CROChrgrRdy_numb/1 -> GcGDP_CROChrgrRdy_numb/1  "GcGDP_CROChrgrRdy_numb"
  Data Type Conversion1/1 -> " CRORecOnce"/2(GeDCC_DCConnSt_enum), Relational Operator/1
  GcISP_2830ChrgrRdy_numb/1 -> GDP_GcGDP_CROChrgrRdy_numb/1  "GcISP_2830ChrgrRdy_numb"

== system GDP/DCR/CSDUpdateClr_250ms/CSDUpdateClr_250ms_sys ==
  Constant : Constant  Value=ASWTYPE_FALSE
  GDP_GbGDP_CSDMsgUpd_flg : AIWAYS_Powertrain_BMS_lib/Signals/OverWrite  OverWrite_Value=CbGDP_CSDMsgUpdOvr_flg  OverWrite_flag=CbGDP_CSDMsgUpdOvrSwt_flg
  Signal Conversion1 : SignalConversion  OverrideOpt=off
  GbGDP_CSDMsgUpd_flg : Outport
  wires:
  GDP_GbGDP_CSDMsgUpd_flg/1 -> GbGDP_CSDMsgUpd_flg/1  "GbGDP_CSDMsgUpd_flg"
  Constant/1 -> Signal Conversion1/1
  Signal Conversion1/1 -> GDP_GbGDP_CSDMsgUpd_flg/1

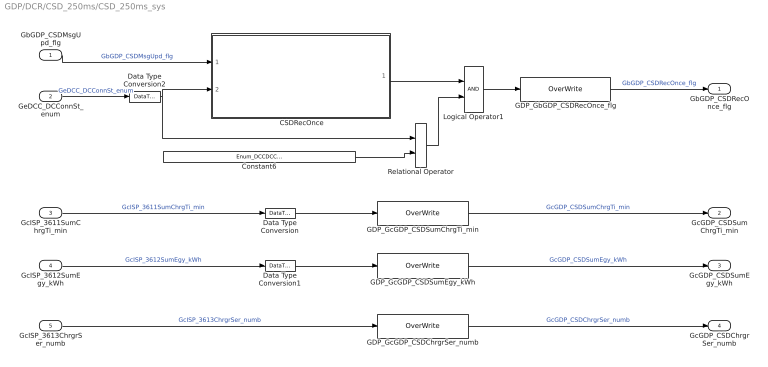
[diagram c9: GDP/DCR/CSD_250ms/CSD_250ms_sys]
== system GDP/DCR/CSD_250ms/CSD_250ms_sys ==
  GbGDP_CSDMsgUpd_flg : Inport
  GeDCC_DCConnSt_enum : Inport  Port=2
  GcISP_3611SumChrgTi_min : Inport  Port=3
  GcISP_3612SumEgy_kWh : Inport  Port=4
  GcISP_3613ChrgrSer_numb : Inport  Port=5
  " CSDRecOnce" : Subsystem
  Constant6 : Constant  Value=Enum_DCCDCConnSt.Enum_DCCDCConnSt_ChrgFin
  Data Type Conversion : DataTypeConversion
  Data Type Conversion1 : DataTypeConversion
  Data Type Conversion2 : DataTypeConversion
  GDP_GbGDP_CSDRecOnce_flg : AIWAYS_Powertrain_BMS_lib/Signals/OverWrite  OverWrite_Value=CbGDP_CSDRecOnceOvr_flg  OverWrite_flag=CbGDP_CSDRecOnceOvrSwt_flg
  GDP_GcGDP_CSDChrgrSer_numb : AIWAYS_Powertrain_BMS_lib/Signals/OverWrite  OverWrite_Value=CcGDP_CSDChrgrSerOvr_numb  OverWrite_flag=CbGDP_CSDChrgrSerOvrSwt_flg
  GDP_GcGDP_CSDSumChrgTi_min : AIWAYS_Powertrain_BMS_lib/Signals/OverWrite  OverWrite_Value=CcGDP_CSDSumChrgTiOvr_min  OverWrite_flag=CbGDP_CSDSumChrgTiOvrSwt_flg
  GDP_GcGDP_CSDSumEgy_kWh : AIWAYS_Powertrain_BMS_lib/Signals/OverWrite  OverWrite_Value=CcGDP_CSDSumEgyOvr_kWh  OverWrite_flag=CbGDP_CSDSumEgyOvrSwt_flg
  Logical Operator1 : Logic  AllPortsSameDT=off  OutDataTypeStr=boolean
  Relational Operator : RelationalOperator  Operator===  OutDataTypeStr=boolean
  GbGDP_CSDRecOnce_flg : Outport
  GcGDP_CSDSumChrgTi_min : Outport  Port=2
  GcGDP_CSDSumEgy_kWh : Outport  Port=3
  GcGDP_CSDChrgrSer_numb : Outport  Port=4
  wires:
  GbGDP_CSDMsgUpd_flg/1 -> " CSDRecOnce"/1(GbGDP_CSDMsgUpd_flg)  "GbGDP_CSDMsgUpd_flg"
  Relational Operator/1 -> Logical Operator1/2
  Constant6/1 -> Relational Operator/2
  " CSDRecOnce"/1(LbGDP_CSDRecOnce_flg) -> Logical Operator1/1
  Logical Operator1/1 -> GDP_GbGDP_CSDRecOnce_flg/1
  GeDCC_DCConnSt_enum/1 -> Data Type Conversion2/1  "GeDCC_DCConnSt_enum"
  GcISP_3611SumChrgTi_min/1 -> Data Type Conversion/1  "GcISP_3611SumChrgTi_min"
  GcISP_3612SumEgy_kWh/1 -> Data Type Conversion1/1  "GcISP_3612SumEgy_kWh"
  GcISP_3613ChrgrSer_numb/1 -> GDP_GcGDP_CSDChrgrSer_numb/1  "GcISP_3613ChrgrSer_numb"
  GDP_GbGDP_CSDRecOnce_flg/1 -> GbGDP_CSDRecOnce_flg/1  "GbGDP_CSDRecOnce_flg"
  GDP_GcGDP_CSDSumChrgTi_min/1 -> GcGDP_CSDSumChrgTi_min/1  "GcGDP_CSDSumChrgTi_min"
  GDP_GcGDP_CSDSumEgy_kWh/1 -> GcGDP_CSDSumEgy_kWh/1  "GcGDP_CSDSumEgy_kWh"
  GDP_GcGDP_CSDChrgrSer_numb/1 -> GcGDP_CSDChrgrSer_numb/1  "GcGDP_CSDChrgrSer_numb"
  Data Type Conversion/1 -> GDP_GcGDP_CSDSumChrgTi_min/1
  Data Type Conversion1/1 -> GDP_GcGDP_CSDSumEgy_kWh/1
  Data Type Conversion2/1 -> " CSDRecOnce"/2(GeDCC_DCConnSt_enum), Relational Operator/1

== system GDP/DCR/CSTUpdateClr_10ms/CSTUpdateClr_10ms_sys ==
  Constant : Constant  Value=ASWTYPE_FALSE
  GDP_GbGDP_CSTMsgUpd_flg : AIWAYS_Powertrain_BMS_lib/Signals/OverWrite  OverWrite_Value=CbGDP_CSTMsgUpdOvr_flg  OverWrite_flag=CbGDP_CSTMsgUpdOvrSwt_flg
  Signal Conversion1 : SignalConversion  OverrideOpt=off
  GbGDP_CSTMsgUpd_flg : Outport
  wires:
  GDP_GbGDP_CSTMsgUpd_flg/1 -> GbGDP_CSTMsgUpd_flg/1  "GbGDP_CSTMsgUpd_flg"
  Constant/1 -> Signal Conversion1/1
  Signal Conversion1/1 -> GDP_GbGDP_CSTMsgUpd_flg/1

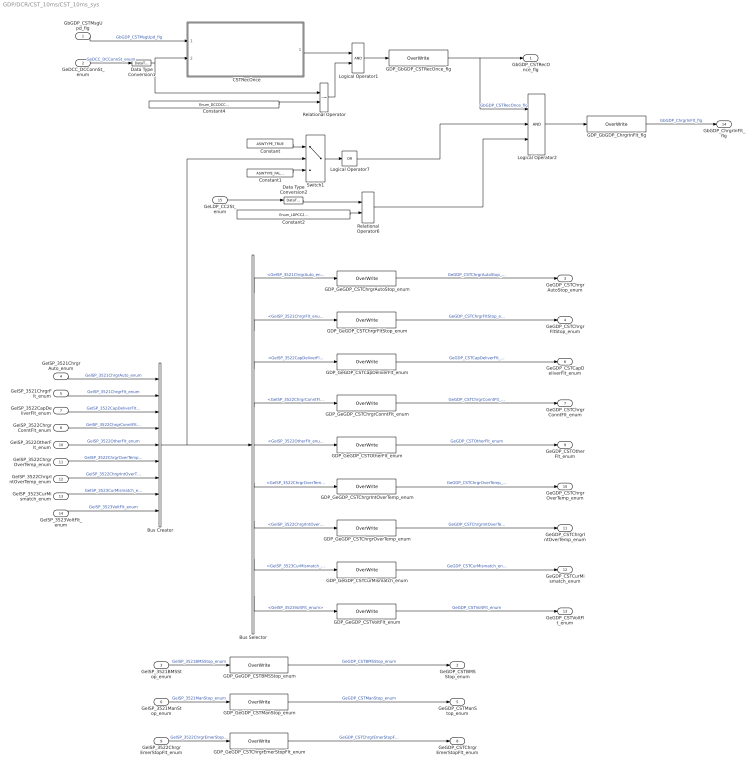
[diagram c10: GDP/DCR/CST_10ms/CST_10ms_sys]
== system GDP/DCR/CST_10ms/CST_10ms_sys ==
  GbGDP_CSTMsgUpd_flg : Inport
  GeDCC_DCConnSt_enum : Inport  Port=2
  GeISP_3521BMSStop_enum : Inport  Port=3
  GeISP_3521ChrgrAuto_enum : Inport  Port=4
  GeISP_3521ChrgrFlt_enum : Inport  Port=5
  GeISP_3521ManStop_enum : Inport  Port=6
  GeISP_3522CapDeliverFlt_enum : Inport  Port=7
  GeISP_3522ChrgrConntFlt_enum : Inport  Port=8
  GeISP_3522ChrgrEmerStopFlt_enum : Inport  Port=9
  GeISP_3522OtherFlt_enum : Inport  Port=10
  GeISP_3522ChrgrOverTemp_enum : Inport  Port=11
  GeISP_3522ChrgrIntOverTemp_enum : Inport  Port=12
  GeISP_3523CurMismatch_enum : Inport  Port=13
  GeISP_3523VoltFlt_enum : Inport  Port=14
  GeLDP_CC2St_enum : Inport  Port=15
  " CSTRecOnce" : Subsystem
  Bus Creator : BusCreator  Inputs=9
  Bus Selector : BusSelector  OutputSignals=GeISP_3521ChrgrAuto_enum,GeISP_3521ChrgrFlt_enum,GeISP_3522CapDeliverFlt_enum,GeISP_3522ChrgrConntFlt_enum,GeISP_3522OtherFlt_enum,GeISP_3522ChrgrOverTemp_enum,GeISP_3522ChrgrIntOverTemp_enum,GeISP_3523CurMismatch_enum,GeISP_3523VoltFlt_enum
  Constant : Constant  Value=ASWTYPE_TRUE
  Constant1 : Constant  Value=ASWTYPE_FALSE
  Constant2 : Constant  Value=Enum_LDPCC2St.Enum_LDPCC2St_Connect
  Constant4 : Constant  Value=Enum_DCCDCConnSt.Enum_DCCDCConnSt_Default
  Data Type Conversion1 : DataTypeConversion
  Data Type Conversion2 : DataTypeConversion
  GDP_GbGDP_CSTRecOnce_flg : AIWAYS_Powertrain_BMS_lib/Signals/OverWrite  OverWrite_Value=CbGDP_CSTRecOnceOvr_flg  OverWrite_flag=CbGDP_CSTRecOnceOvrSwt_flg
  GDP_GbGDP_ChrgrInFlt_flg : AIWAYS_Powertrain_BMS_lib/Signals/OverWrite  OverWrite_Value=CbGDP_ChrgrInFltOvr_flg  OverWrite_flag=CbGDP_ChrgrInFltOvrSwt_flg
  GDP_GeGDP_CSTBMSStop_enum : AIWAYS_Powertrain_BMS_lib/Signals/OverWrite  OverWrite_Value=CeGDP_CSTBMSStopOvr_enum  OverWrite_flag=CbGDP_CSTBMSStopOvrSwt_flg
  GDP_GeGDP_CSTCapDeliverFlt_enum : AIWAYS_Powertrain_BMS_lib/Signals/OverWrite  OverWrite_Value=CeGDP_CSTCapDeliverFltOvr_enum  OverWrite_flag=CbGDP_CSTCapDeliverFltOvrSwt_flg
  GDP_GeGDP_CSTChrgrAutoStop_enum : AIWAYS_Powertrain_BMS_lib/Signals/OverWrite  OverWrite_Value=CeGDP_CSTChrgrAutoStopOvr_enum  OverWrite_flag=CbGDP_CSTChrgrAutoStopOvrSwt_flg
  GDP_GeGDP_CSTChrgrConntFlt_enum : AIWAYS_Powertrain_BMS_lib/Signals/OverWrite  OverWrite_Value=CeGDP_CSTChrgrConntFltOvr_enum  OverWrite_flag=CbGDP_CSTChrgrConntFltOvrSwt_flg
  GDP_GeGDP_CSTChrgrEmerStopFlt_enum : AIWAYS_Powertrain_BMS_lib/Signals/OverWrite  OverWrite_Value=CeGDP_CSTChrgrEmerStopFltOvr_enum  OverWrite_flag=CbGDP_CSTChrgrEmerStopFltOvrSwt_flg
  GDP_GeGDP_CSTChrgrFltStop_enum : AIWAYS_Powertrain_BMS_lib/Signals/OverWrite  OverWrite_Value=CeGDP_CSTChrgrFltStopOvr_enum  OverWrite_flag=CbGDP_CSTChrgrFltStopOvrSwt_flg
  GDP_GeGDP_CSTChrgrIntOverTemp_enum : AIWAYS_Powertrain_BMS_lib/Signals/OverWrite  OverWrite_Value=CeGDP_CSTChrgrOverTempOvr_enum  OverWrite_flag=CbGDP_CSTChrgrOverTempOvrSwt_flg
  GDP_GeGDP_CSTChrgrOverTemp_enum : AIWAYS_Powertrain_BMS_lib/Signals/OverWrite  OverWrite_Value=CeGDP_CSTChrgrIntOverTempOvr_enum  OverWrite_flag=CbGDP_CSTChrgrIntOverTempOvrSwt_flg
  GDP_GeGDP_CSTCurMismatch_enum : AIWAYS_Powertrain_BMS_lib/Signals/OverWrite  OverWrite_Value=CeGDP_CSTCurMismatchOvr_enum  OverWrite_flag=CbGDP_CSTCurMismatchOvrSwt_flg
  GDP_GeGDP_CSTManStop_enum : AIWAYS_Powertrain_BMS_lib/Signals/OverWrite  OverWrite_Value=CeGDP_CSTManStopOvr_enum  OverWrite_flag=CbGDP_CSTManStopOvrSwt_flg
  GDP_GeGDP_CSTOtherFlt_enum : AIWAYS_Powertrain_BMS_lib/Signals/OverWrite  OverWrite_Value=CeGDP_CSTOtherFltOvr_enum  OverWrite_flag=CbGDP_CSTOtherFltOvrSwt_flg
  GDP_GeGDP_CSTVoltFlt_enum : AIWAYS_Powertrain_BMS_lib/Signals/OverWrite  OverWrite_Value=CeGDP_CSTVoltFltOvr_enum  OverWrite_flag=CbGDP_CSTVoltFltOvrSwt_flg
  Logical Operator1 : Logic  AllPortsSameDT=off  OutDataTypeStr=boolean
  Logical Operator2 : Logic  Inputs=3  AllPortsSameDT=off  OutDataTypeStr=boolean
  Logical Operator7 : Logic  Operator=OR  Inputs=1  AllPortsSameDT=off  OutDataTypeStr=boolean
  Relational Operator : RelationalOperator  Operator=~=  OutDataTypeStr=boolean
  Relational Operator6 : RelationalOperator  Operator===  OutDataTypeStr=boolean
  Switch1 : Switch  Criteria=u2 ~= 0
  GbGDP_CSTRecOnce_flg : Outport
  GeGDP_CSTBMSStop_enum : Outport  Port=2
  GeGDP_CSTChrgrAutoStop_enum : Outport  Port=3
  GeGDP_CSTChrgrFltStop_enum : Outport  Port=4
  GeGDP_CSTManStop_enum : Outport  Port=5
  GeGDP_CSTCapDeliverFlt_enum : Outport  Port=6
  GeGDP_CSTChrgrConntFlt_enum : Outport  Port=7
  GeGDP_CSTChrgrEmerStopFlt_enum : Outport  Port=8
  GeGDP_CSTOtherFlt_enum : Outport  Port=9
  GeGDP_CSTChrgrOverTemp_enum : Outport  Port=10
  GeGDP_CSTChrgrIntOverTemp_enum : Outport  Port=11
  GeGDP_CSTCurMismatch_enum : Outport  Port=12
  GeGDP_CSTVoltFlt_enum : Outport  Port=13
  GbGDP_ChrgrInFlt_flg : Outport  Port=14
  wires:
  GbGDP_CSTMsgUpd_flg/1 -> " CSTRecOnce"/1(GbGDP_CSTMsgUpd_flg)  "GbGDP_CSTMsgUpd_flg"
  Relational Operator/1 -> Logical Operator1/2
  Constant4/1 -> Relational Operator/2
  " CSTRecOnce"/1(LbGDP_CSTRecOnce_flg) -> Logical Operator1/1
  Logical Operator1/1 -> GDP_GbGDP_CSTRecOnce_flg/1
  GeDCC_DCConnSt_enum/1 -> Data Type Conversion1/1  "GeDCC_DCConnSt_enum"
  GDP_GbGDP_CSTRecOnce_flg/1 -> Logical Operator2/1, GbGDP_CSTRecOnce_flg/1  "GbGDP_CSTRecOnce_flg"
  GDP_GeGDP_CSTChrgrAutoStop_enum/1 -> GeGDP_CSTChrgrAutoStop_enum/1  "GeGDP_CSTChrgrAutoStop_enum"
  GDP_GeGDP_CSTBMSStop_enum/1 -> GeGDP_CSTBMSStop_enum/1  "GeGDP_CSTBMSStop_enum"
  GDP_GeGDP_CSTChrgrFltStop_enum/1 -> GeGDP_CSTChrgrFltStop_enum/1  "GeGDP_CSTChrgrFltStop_enum"
  GDP_GeGDP_CSTManStop_enum/1 -> GeGDP_CSTManStop_enum/1  "GeGDP_CSTManStop_enum"
  GDP_GeGDP_CSTCapDeliverFlt_enum/1 -> GeGDP_CSTCapDeliverFlt_enum/1  "GeGDP_CSTCapDeliverFlt_enum"
  GDP_GeGDP_CSTChrgrConntFlt_enum/1 -> GeGDP_CSTChrgrConntFlt_enum/1  "GeGDP_CSTChrgrConntFlt_enum"
  GDP_GeGDP_CSTChrgrEmerStopFlt_enum/1 -> GeGDP_CSTChrgrEmerStopFlt_enum/1  "GeGDP_CSTChrgrEmerStopFlt_enum"
  GDP_GeGDP_CSTOtherFlt_enum/1 -> GeGDP_CSTOtherFlt_enum/1  "GeGDP_CSTOtherFlt_enum"
  GDP_GeGDP_CSTCurMismatch_enum/1 -> GeGDP_CSTCurMismatch_enum/1  "GeGDP_CSTCurMismatch_enum"
  GDP_GeGDP_CSTVoltFlt_enum/1 -> GeGDP_CSTVoltFlt_enum/1  "GeGDP_CSTVoltFlt_enum"
  GDP_GeGDP_CSTChrgrIntOverTemp_enum/1 -> GeGDP_CSTChrgrOverTemp_enum/1  "GeGDP_CSTChrgrOverTemp_enum"
  GDP_GeGDP_CSTChrgrOverTemp_enum/1 -> GeGDP_CSTChrgrIntOverTemp_enum/1  "GeGDP_CSTChrgrIntOverTemp_enum"
  GeISP_3521ChrgrAuto_enum/1 -> Bus Creator/1  "GeISP_3521ChrgrAuto_enum"
  GeISP_3521ChrgrFlt_enum/1 -> Bus Creator/2  "GeISP_3521ChrgrFlt_enum"
  GeISP_3522CapDeliverFlt_enum/1 -> Bus Creator/3  "GeISP_3522CapDeliverFlt_enum"
  GeISP_3522ChrgrConntFlt_enum/1 -> Bus Creator/4  "GeISP_3522ChrgrConntFlt_enum"
  GeISP_3522OtherFlt_enum/1 -> Bus Creator/5  "GeISP_3522OtherFlt_enum"
  GeISP_3522ChrgrOverTemp_enum/1 -> Bus Creator/6  "GeISP_3522ChrgrOverTemp_enum"
  GeISP_3522ChrgrIntOverTemp_enum/1 -> Bus Creator/7  "GeISP_3522ChrgrIntOverTemp_enum"
  GeISP_3523CurMismatch_enum/1 -> Bus Creator/8  "GeISP_3523CurMismatch_enum"
  GeISP_3523VoltFlt_enum/1 -> Bus Creator/9  "GeISP_3523VoltFlt_enum"
  Bus Selector/1 -> GDP_GeGDP_CSTChrgrAutoStop_enum/1  "<GeISP_3521ChrgrAuto_enum>"
  Bus Selector/2 -> GDP_GeGDP_CSTChrgrFltStop_enum/1  "<GeISP_3521ChrgrFlt_enum>"
  Bus Selector/3 -> GDP_GeGDP_CSTCapDeliverFlt_enum/1  "<GeISP_3522CapDeliverFlt_enum>"
  Bus Selector/4 -> GDP_GeGDP_CSTChrgrConntFlt_enum/1  "<GeISP_3522ChrgrConntFlt_enum>"
  Bus Selector/5 -> GDP_GeGDP_CSTOtherFlt_enum/1  "<GeISP_3522OtherFlt_enum>"
  Bus Selector/6 -> GDP_GeGDP_CSTChrgrIntOverTemp_enum/1  "<GeISP_3522ChrgrOverTemp_enum>"
  Bus Selector/7 -> GDP_GeGDP_CSTChrgrOverTemp_enum/1  "<GeISP_3522ChrgrIntOverTemp_enum>"
  Bus Selector/8 -> GDP_GeGDP_CSTCurMismatch_enum/1  "<GeISP_3523CurMismatch_enum>"
  Bus Selector/9 -> GDP_GeGDP_CSTVoltFlt_enum/1  "<GeISP_3523VoltFlt_enum>"
  GeISP_3521BMSStop_enum/1 -> GDP_GeGDP_CSTBMSStop_enum/1  "GeISP_3521BMSStop_enum"
  GeISP_3522ChrgrEmerStopFlt_enum/1 -> GDP_GeGDP_CSTChrgrEmerStopFlt_enum/1  "GeISP_3522ChrgrEmerStopFlt_enum"
  GeISP_3521ManStop_enum/1 -> GDP_GeGDP_CSTManStop_enum/1  "GeISP_3521ManStop_enum"
  Constant1/1 -> Switch1/3
  Bus Creator/1 -> Bus Selector/1, Switch1/2
  Constant/1 -> Switch1/1
  Switch1/1 -> Logical Operator7/1
  GDP_GbGDP_ChrgrInFlt_flg/1 -> GbGDP_ChrgrInFlt_flg/1  "GbGDP_ChrgrInFlt_flg"
  Data Type Conversion1/1 -> " CSTRecOnce"/2(GeDCC_DCConnSt_enum), Relational Operator/1
  GeLDP_CC2St_enum/1 -> Data Type Conversion2/1
  Constant2/1 -> Relational Operator6/2
  Data Type Conversion2/1 -> Relational Operator6/1
  Logical Operator2/1 -> GDP_GbGDP_ChrgrInFlt_flg/1
  Logical Operator7/1 -> Logical Operator2/2
  Relational Operator6/1 -> Logical Operator2/3

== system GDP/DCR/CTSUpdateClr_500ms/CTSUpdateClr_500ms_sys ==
  Constant : Constant  Value=ASWTYPE_FALSE
  GDP_GbGDP_CTSMsgUpd_flg : AIWAYS_Powertrain_BMS_lib/Signals/OverWrite  OverWrite_Value=CbGDP_CTSMsgUpdOvr_flg  OverWrite_flag=CbGDP_CTSMsgUpdOvrSwt_flg
  Signal Conversion1 : SignalConversion  OverrideOpt=off
  GbGDP_CTSMsgUpd_flg : Outport
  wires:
  Signal Conversion1/1 -> GDP_GbGDP_CTSMsgUpd_flg/1
  GDP_GbGDP_CTSMsgUpd_flg/1 -> GbGDP_CTSMsgUpd_flg/1  "GbGDP_CTSMsgUpd_flg"
  Constant/1 -> Signal Conversion1/1

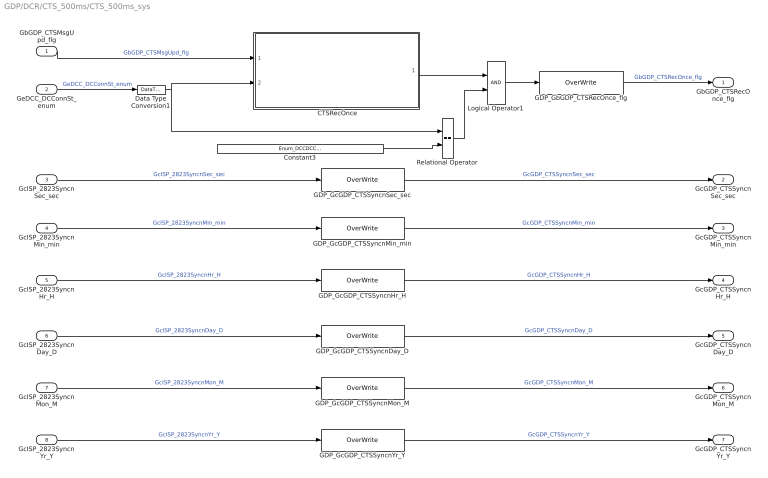
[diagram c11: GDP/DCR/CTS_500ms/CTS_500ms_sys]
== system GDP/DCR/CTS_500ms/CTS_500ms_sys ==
  GbGDP_CTSMsgUpd_flg : Inport
  GeDCC_DCConnSt_enum : Inport  Port=2
  GcISP_2823SyncnSec_sec : Inport  Port=3
  GcISP_2823SyncnMin_min : Inport  Port=4
  GcISP_2823SyncnHr_H : Inport  Port=5
  GcISP_2823SyncnDay_D : Inport  Port=6
  GcISP_2823SyncnMon_M : Inport  Port=7
  GcISP_2823SyncnYr_Y : Inport  Port=8
  " CTSRecOnce" : Subsystem
  Constant3 : Constant  Value=Enum_DCCDCConnSt.Enum_DCCDCConnSt_CFG
  Data Type Conversion1 : DataTypeConversion
  GDP_GbGDP_CTSRecOnce_flg : AIWAYS_Powertrain_BMS_lib/Signals/OverWrite  OverWrite_Value=CbGDP_CTSRecOnceOvr_flg  OverWrite_flag=CbGDP_CTSRecOnceOvrSwt_flg
  GDP_GcGDP_CTSSyncnDay_D : AIWAYS_Powertrain_BMS_lib/Signals/OverWrite  OverWrite_Value=CcGDP_CTSSyncnDayOvr_D  OverWrite_flag=CbGDP_CTSSyncnDayOvrSwt_flg
  GDP_GcGDP_CTSSyncnHr_H : AIWAYS_Powertrain_BMS_lib/Signals/OverWrite  OverWrite_Value=CcGDP_CTSSyncnHrOvr_H  OverWrite_flag=CbGDP_CTSSyncnHrOvrSwt_flg
  GDP_GcGDP_CTSSyncnMin_min : AIWAYS_Powertrain_BMS_lib/Signals/OverWrite  OverWrite_Value=CcGDP_CTSSyncnMinOvr_min  OverWrite_flag=CbGDP_CTSSyncnMinOvrSwt_flg
  GDP_GcGDP_CTSSyncnMon_M : AIWAYS_Powertrain_BMS_lib/Signals/OverWrite  OverWrite_Value=CcGDP_CTSSyncnMonOvr_M  OverWrite_flag=CbGDP_CTSSyncnMonOvrSwt_flg
  GDP_GcGDP_CTSSyncnSec_sec : AIWAYS_Powertrain_BMS_lib/Signals/OverWrite  OverWrite_Value=CcGDP_CTSSyncnSecOvr_sec  OverWrite_flag=CbGDP_CTSSyncnSecOvrSwt_flg
  GDP_GcGDP_CTSSyncnYr_Y : AIWAYS_Powertrain_BMS_lib/Signals/OverWrite  OverWrite_Value=CcGDP_CTSSyncnYrOvr_Y  OverWrite_flag=CbGDP_CTSSyncnYrOvrSwt_flg
  Logical Operator1 : Logic  AllPortsSameDT=off  OutDataTypeStr=boolean
  Relational Operator : RelationalOperator  Operator===  OutDataTypeStr=boolean
  GbGDP_CTSRecOnce_flg : Outport
  GcGDP_CTSSyncnSec_sec : Outport  Port=2
  GcGDP_CTSSyncnMin_min : Outport  Port=3
  GcGDP_CTSSyncnHr_H : Outport  Port=4
  GcGDP_CTSSyncnDay_D : Outport  Port=5
  GcGDP_CTSSyncnMon_M : Outport  Port=6
  GcGDP_CTSSyncnYr_Y : Outport  Port=7
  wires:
  GbGDP_CTSMsgUpd_flg/1 -> " CTSRecOnce"/1(GbGDP_CTSMsgUpd_flg)  "GbGDP_CTSMsgUpd_flg"
  Relational Operator/1 -> Logical Operator1/2
  Constant3/1 -> Relational Operator/2
  " CTSRecOnce"/1(LbGDP_CTSRecOnce_flg) -> Logical Operator1/1
  Logical Operator1/1 -> GDP_GbGDP_CTSRecOnce_flg/1
  GeDCC_DCConnSt_enum/1 -> Data Type Conversion1/1  "GeDCC_DCConnSt_enum"
  GcISP_2823SyncnSec_sec/1 -> GDP_GcGDP_CTSSyncnSec_sec/1  "GcISP_2823SyncnSec_sec"
  GcISP_2823SyncnMin_min/1 -> GDP_GcGDP_CTSSyncnMin_min/1  "GcISP_2823SyncnMin_min"
  GcISP_2823SyncnYr_Y/1 -> GDP_GcGDP_CTSSyncnYr_Y/1  "GcISP_2823SyncnYr_Y"
  GcISP_2823SyncnMon_M/1 -> GDP_GcGDP_CTSSyncnMon_M/1  "GcISP_2823SyncnMon_M"
  GcISP_2823SyncnDay_D/1 -> GDP_GcGDP_CTSSyncnDay_D/1  "GcISP_2823SyncnDay_D"
  GcISP_2823SyncnHr_H/1 -> GDP_GcGDP_CTSSyncnHr_H/1  "GcISP_2823SyncnHr_H"
  GDP_GbGDP_CTSRecOnce_flg/1 -> GbGDP_CTSRecOnce_flg/1  "GbGDP_CTSRecOnce_flg"
  GDP_GcGDP_CTSSyncnSec_sec/1 -> GcGDP_CTSSyncnSec_sec/1  "GcGDP_CTSSyncnSec_sec"
  GDP_GcGDP_CTSSyncnMin_min/1 -> GcGDP_CTSSyncnMin_min/1  "GcGDP_CTSSyncnMin_min"
  GDP_GcGDP_CTSSyncnHr_H/1 -> GcGDP_CTSSyncnHr_H/1  "GcGDP_CTSSyncnHr_H"
  GDP_GcGDP_CTSSyncnDay_D/1 -> GcGDP_CTSSyncnDay_D/1  "GcGDP_CTSSyncnDay_D"
  GDP_GcGDP_CTSSyncnMon_M/1 -> GcGDP_CTSSyncnMon_M/1  "GcGDP_CTSSyncnMon_M"
  GDP_GcGDP_CTSSyncnYr_Y/1 -> GcGDP_CTSSyncnYr_Y/1  "GcGDP_CTSSyncnYr_Y"
  Data Type Conversion1/1 -> " CTSRecOnce"/2(GeDCC_DCConnSt_enum), Relational Operator/1

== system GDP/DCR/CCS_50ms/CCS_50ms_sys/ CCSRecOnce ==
  GbGDP_CCSMsgUpd_flg : Inport
  GeDCC_DCConnSt_enum : Inport  Port=2
  CCSMsg : Subsystem
  Constant5 : Constant  Value=Enum_DCCDCConnSt.Enum_DCCDCConnSt_Chrging
  Relational Operator : RelationalOperator  Operator===  OutDataTypeStr=boolean
  LbGDP_CCSRecOnce_flg : Outport
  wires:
  GeDCC_DCConnSt_enum/1 -> Relational Operator/1
  Constant5/1 -> Relational Operator/2
  GbGDP_CCSMsgUpd_flg/1 -> CCSMsg/1(GbGDP_CCSMsgUpd_flg)
  CCSMsg/1(LbGDP_CCSRecOnce_flg) -> LbGDP_CCSRecOnce_flg/1
  Relational Operator/1 -> CCSMsg/Enable

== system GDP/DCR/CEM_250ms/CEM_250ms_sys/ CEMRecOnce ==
  GbGDP_CEMMsgUpd_flg : Inport
  GeDCC_DCConnSt_enum : Inport  Port=2
  CEMMsg : Subsystem
  Constant4 : Constant  Value=Enum_DCCDCConnSt.Enum_DCCDCConnSt_Default
  Relational Operator : RelationalOperator  Operator=~=  OutDataTypeStr=boolean
  LbGDP_CEMRecOnce_flg : Outport
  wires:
  GeDCC_DCConnSt_enum/1 -> Relational Operator/1
  Constant4/1 -> Relational Operator/2
  GbGDP_CEMMsgUpd_flg/1 -> CEMMsg/1(GbGDP_CEMMsgUpd_flg)
  CEMMsg/1(LbGDP_CEMRecOnce_flg) -> LbGDP_CEMRecOnce_flg/1
  Relational Operator/1 -> CEMMsg/Enable

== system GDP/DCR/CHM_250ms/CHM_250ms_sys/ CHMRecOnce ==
  GbGDP_CHMMsgUpd_flg : Inport
  GbLDP_DC12VSply_flg : Inport  Port=2
  GeDCC_DCConnSt_enum : Inport  Port=3
  CHMMsg : Subsystem
  Constant1 : Constant  Value=Enum_DCCDCConnSt.Enum_DCCDCConnSt_HandShake
  Constant4 : Constant  Value=Enum_DCCDCConnSt.Enum_DCCDCConnSt_Default
  Logical Operator : Logic  Operator=OR  AllPortsSameDT=off  OutDataTypeStr=boolean
  Logical Operator1 : Logic  AllPortsSameDT=off  OutDataTypeStr=boolean
  Relational Operator : RelationalOperator  Operator===  OutDataTypeStr=boolean
  Relational Operator1 : RelationalOperator  Operator===  OutDataTypeStr=boolean
  LbGDP_CHMRecOnce_flg : Outport
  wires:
  Constant1/1 -> Relational Operator1/2
  Constant4/1 -> Relational Operator/2
  Relational Operator/1 -> Logical Operator/1
  Relational Operator1/1 -> Logical Operator/2
  GbGDP_CHMMsgUpd_flg/1 -> CHMMsg/1(GbGDP_CHMMsgUpd_flg)
  CHMMsg/1(LbGDP_CHMRecOnce_flg) -> LbGDP_CHMRecOnce_flg/1
  GeDCC_DCConnSt_enum/1 -> Relational Operator/1, Relational Operator1/1
  GbLDP_DC12VSply_flg/1 -> Logical Operator1/2
  Logical Operator/1 -> Logical Operator1/1
  Logical Operator1/1 -> CHMMsg/Enable

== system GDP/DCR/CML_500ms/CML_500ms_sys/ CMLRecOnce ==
  GbGDP_CMLMsgUpd_flg : Inport
  GeDCC_DCConnSt_enum : Inport  Port=2
  CMLMsg : Subsystem
  Constant3 : Constant  Value=Enum_DCCDCConnSt.Enum_DCCDCConnSt_CFG
  Relational Operator : RelationalOperator  Operator===  OutDataTypeStr=boolean
  LbGDP_CMLRecOnce_flg : Outport
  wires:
  GbGDP_CMLMsgUpd_flg/1 -> CMLMsg/1(GbGDP_CMLMsgUpd_flg)
  CMLMsg/1(LbGDP_CMLRecOnce_flg) -> LbGDP_CMLRecOnce_flg/1
  Relational Operator/1 -> CMLMsg/Enable
  Constant3/1 -> Relational Operator/2
  GeDCC_DCConnSt_enum/1 -> Relational Operator/1

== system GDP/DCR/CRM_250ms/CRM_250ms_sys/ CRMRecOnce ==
  GbGDP_CRMMsgUpd_flg : Inport
  GeDCC_DCConnSt_enum : Inport  Port=2
  CRMMsg : Subsystem
  Constant1 : Constant  Value=Enum_DCCDCConnSt.Enum_DCCDCConnSt_HandShake
  Constant2 : Constant  Value=Enum_DCCDCConnSt.Enum_DCCDCConnSt_ID
  Constant3 : Constant  Value=Enum_DCCDCConnSt.Enum_DCCDCConnSt_CommTout
  Logical Operator : Logic  Operator=OR  Inputs=3  AllPortsSameDT=off  OutDataTypeStr=boolean
  Relational Operator : RelationalOperator  Operator===  OutDataTypeStr=boolean
  Relational Operator1 : RelationalOperator  Operator===  OutDataTypeStr=boolean
  Relational Operator2 : RelationalOperator  Operator===  OutDataTypeStr=boolean
  LbGDP_CRMRecOnce_flg : Outport
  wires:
  GeDCC_DCConnSt_enum/1 -> Relational Operator2/1, Relational Operator1/1, Relational Operator/1
  Constant1/1 -> Relational Operator1/2
  Constant2/1 -> Relational Operator/2
  Relational Operator/1 -> Logical Operator/1
  Relational Operator1/1 -> Logical Operator/2
  GbGDP_CRMMsgUpd_flg/1 -> CRMMsg/1(GbGDP_CRMMsgUpd_flg)
  CRMMsg/1(LbGDP_CRMRecOnce_flg) -> LbGDP_CRMRecOnce_flg/1
  Logical Operator/1 -> CRMMsg/Enable
  Constant3/1 -> Relational Operator2/2
  Relational Operator2/1 -> Logical Operator/3

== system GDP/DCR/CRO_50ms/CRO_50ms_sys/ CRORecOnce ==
  GbGDP_CROMsgUpd_flg : Inport
  GeDCC_DCConnSt_enum : Inport  Port=2
  CROMsg : Subsystem
  Constant3 : Constant  Value=Enum_DCCDCConnSt.Enum_DCCDCConnSt_CFG
  Relational Operator : RelationalOperator  Operator===  OutDataTypeStr=boolean
  LbGDP_CRORecOnce_flg : Outport
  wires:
  Relational Operator/1 -> CROMsg/Enable
  GeDCC_DCConnSt_enum/1 -> Relational Operator/1
  Constant3/1 -> Relational Operator/2
  GbGDP_CROMsgUpd_flg/1 -> CROMsg/1(GbGDP_CROMsgUpd_flg)
  CROMsg/1(LbGDP_CRORecOnce_flg) -> LbGDP_CRORecOnce_flg/1

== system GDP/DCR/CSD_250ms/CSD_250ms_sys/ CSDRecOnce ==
  GbGDP_CSDMsgUpd_flg : Inport
  GeDCC_DCConnSt_enum : Inport  Port=2
  CSDMsg : Subsystem
  Constant6 : Constant  Value=Enum_DCCDCConnSt.Enum_DCCDCConnSt_ChrgFin
  Relational Operator : RelationalOperator  Operator===  OutDataTypeStr=boolean
  LbGDP_CSDRecOnce_flg : Outport
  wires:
  GeDCC_DCConnSt_enum/1 -> Relational Operator/1
  Constant6/1 -> Relational Operator/2
  GbGDP_CSDMsgUpd_flg/1 -> CSDMsg/1(GbGDP_CSDMsgUpd_flg)
  CSDMsg/1(LbGDP_CSDRecOnce_flg) -> LbGDP_CSDRecOnce_flg/1
  Relational Operator/1 -> CSDMsg/Enable

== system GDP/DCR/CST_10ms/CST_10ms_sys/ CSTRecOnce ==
  GbGDP_CSTMsgUpd_flg : Inport
  GeDCC_DCConnSt_enum : Inport  Port=2
  CSTMsg : Subsystem
  Constant4 : Constant  Value=Enum_DCCDCConnSt.Enum_DCCDCConnSt_Default
  Relational Operator : RelationalOperator  Operator=~=  OutDataTypeStr=boolean
  LbGDP_CSTRecOnce_flg : Outport
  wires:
  Relational Operator/1 -> CSTMsg/Enable
  GeDCC_DCConnSt_enum/1 -> Relational Operator/1
  Constant4/1 -> Relational Operator/2
  GbGDP_CSTMsgUpd_flg/1 -> CSTMsg/1(GbGDP_CSTMsgUpd_flg)
  CSTMsg/1(LbGDP_CSTRecOnce_flg) -> LbGDP_CSTRecOnce_flg/1

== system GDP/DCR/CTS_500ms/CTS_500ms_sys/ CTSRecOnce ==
  GbGDP_CTSMsgUpd_flg : Inport
  GeDCC_DCConnSt_enum : Inport  Port=2
  CTSMsg : Subsystem
  Constant3 : Constant  Value=Enum_DCCDCConnSt.Enum_DCCDCConnSt_CFG
  Relational Operator : RelationalOperator  Operator===  OutDataTypeStr=boolean
  LbGDP_CTSRecOnce_flg : Outport
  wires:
  GeDCC_DCConnSt_enum/1 -> Relational Operator/1
  Constant3/1 -> Relational Operator/2
  GbGDP_CTSMsgUpd_flg/1 -> CTSMsg/1(GbGDP_CTSMsgUpd_flg)
  CTSMsg/1(LbGDP_CTSRecOnce_flg) -> LbGDP_CTSRecOnce_flg/1
  Relational Operator/1 -> CTSMsg/Enable

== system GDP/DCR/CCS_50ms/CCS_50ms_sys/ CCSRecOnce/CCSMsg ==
  GbGDP_CCSMsgUpd_flg : Inport
  Enable : EnablePort  StatesWhenEnabling=reset
  Logical Operator2 : Logic  Operator=OR  AllPortsSameDT=off  OutDataTypeStr=boolean
  Unit Delay : UnitDelay  SampleTime=-1  StateName=StateName
  LbGDP_CCSRecOnce_flg : Outport
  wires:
  Logical Operator2/1 -> LbGDP_CCSRecOnce_flg/1, Unit Delay/1  "LbGDP_CCSRecOnce_flg"
  GbGDP_CCSMsgUpd_flg/1 -> Logical Operator2/1
  Unit Delay/1 -> Logical Operator2/2

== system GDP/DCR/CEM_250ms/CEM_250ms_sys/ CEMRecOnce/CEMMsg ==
  GbGDP_CEMMsgUpd_flg : Inport
  Enable : EnablePort  StatesWhenEnabling=reset
  Logical Operator2 : Logic  Operator=OR  AllPortsSameDT=off  OutDataTypeStr=boolean
  Unit Delay : UnitDelay  SampleTime=-1  StateName=StateName
  LbGDP_CEMRecOnce_flg : Outport
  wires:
  Logical Operator2/1 -> LbGDP_CEMRecOnce_flg/1, Unit Delay/1  "LbGDP_CEMRecOnce_flg"
  GbGDP_CEMMsgUpd_flg/1 -> Logical Operator2/1
  Unit Delay/1 -> Logical Operator2/2
